| IBIS file 3599z.ibs created by s2ibis2 version 1.1
| North Carolina State University Electronics Research Laboratory  1995
[IBIS ver]   2.1
[File name]   idt70v3599dr.ibs
[File Rev]   2.0
|1.0 : Original Version - Wei-Ling Chang
|2.0 : Replaced I/O and Input models with 70V659 ADC models - S.Kashyap 06/30/04
|3.0:  Modified for DR package - T. Hiatt 4/27/06
[Source]   Integrated Device Technology, Inc.
[Notes]   1.Temperatures: typ=25C, min=100C, max=0C 2.RRmp rates based
   on 50 ohm load. 3. Both inpad and iopad have 2 models each.
   (JTAG pins have one model.)
   iopad: standard 3.3V I/O model
   inpad: standard 3.3V input pad model
   iopad25: For 2.5V I/O supply
   inpad25: For 2.5V I/O supply.
   To use 2.%V models at any port, use iopad25 and inpad25
   as the model definition in pin defie section of the IBIS
   file.  JTAG pins only have models for 3.3V I/O voltage.
[Disclaimer] Integrated Device Technology, Inc. ("IDT") hereby grants the
   user of this IBIS model a non-exclusive, nontransferable
   license to use this IBIS model under the following terms. The
   user is granted this license only to use the IBIS model and is
   not granted rights to sell, copy (except as needed to run the
   IBIS model), rent, lease or sub-license the IBIS model in
   whole or in part, or in modified form to anyone. The User may
   modify the IBIS model to suit its specific applications, but
   rights to derivative works and such modifications shall belong
   to IDT. This IBIS model is provided on an AS IS" basis and IDT
   makes absolutely no warranty with respect to the information
   contained herein. IDT DISCLAIMS AND CUSTOMER WAIVES ALL
   WARRANTIES, EXPRESS AND IMPLIED, INCLUDING WARRANTIES OF
   MERCHANTABILITY AND FITNESS FOR A PARTICULAR PURPOSE. THE
   ENTIRE RISK AS TO QUALITY AND PERFORMANCE IS WITH THE USER
   ACCORDINGLY, IN NO EVENT SHALL IDT BE LIABLE FOR ANY DIRECT OR
   INDIRECT DAMAGES, WHETHER IN CONTRACT OR TORT, INCLUDING ANY
   LOST PROFITS OR OTHER INCIDENTAL, CONSEQUENTIAL, EXEMPLARY, OR
   PUNITIVE DAMAGES ARISING OUT OF THE USE OR APPLICATION OF THE
   IBIS model. Further, IDT reserves the right to make changes
   without notice to any product herein to improve reliability,
   function, or design. IDT does not convey any license under
   patent rights or any other intellectual property rights,
   including those of third parties. IDT is not obligated to
   provide maintenance or support for the licensed IBIS model.
[Copyright]   Copyright 2004, Integrated Device Technology, Inc. all rights
   reserved
|   Component idt70v3599z
[Component]   idt70v3599z
[Manufacturer]   Integrated Device Technology
[Package]
| TQFP (DR208)
| variable   typ   min   max
R_pkg   100.00m   50.00m   0.30
L_pkg   12.00nH   10.00nH   14.00nH
C_pkg   2.80pF   1.50pF   6.00pF
[Pin]  signal_name   model_name   R_pin   L_pin   C_pin
1   io19l   iopad
2   io19r   iopad
3   io20l   iopad
4   io20r   iopad
5   VDDQ   POWER
6   GND   GND
7   io21l   iopad
8   io21r   iopad
9   io22l   iopad
10   io22r   iopad
11   VDDQ   POWER
12   GND   GND
13   io23l   iopad
14   io23r   iopad
15   io24l   iopad
16   io24r   iopad
17   VDDQ   POWER
18   GND   GND
19   io25l   iopad
20   io25r   iopad
21   io26l   iopad
22   io26r   iopad
23   VDDQ   POWER
24   GND   GND
25   VDD   POWER
26   VDD   POWER
27   GND   GND
28   GND   GND
29   VDDQ   POWER
30   GND   GND
31   io27r   iopad
32   io27l   iopad
33   io28r   iopad
34   io28l   iopad
35   VDDQ   POWER
36   GND   GND
37   io29r   iopad
38   io29l   iopad
39   io30r   iopad
40   io30l   iopad
41   VDDQ   POWER
42   GND   GND
43   io31r   iopad
44   io31l   iopad
45   io32r   iopad
46   io32l   iopad
47   VDDQ   POWER
48   GND   GND
49   io33r   iopad
50   io33l   iopad
51   io34r   iopad
52   io34l   iopad
53   GND   GND
54   VDDQ   POWER
55   io35r   iopad
56   io35l   iopad
57   plftr#   inpad
64   a16r   inpad
65   a15r   inpad
66   a14r   inpad
67   a13r   inpad
68   a12r   inpad
69   a11r   inpad
70   a10r   inpad
71   a9r   inpad
72   a8r   inpad
73   a7r   inpad
74   be3r#   inpad
75   be2r#   inpad
76   be1r#   inpad
77   be0r#   inpad
78   ce1r   inpad
79   ce0r   inpad
80   VDD   POWER
81   VDD   POWER
82   GND   GND
83   GND   GND
84   clkr   inpad
85   oe#   inpad
86   rwr#   inpad
87   adsr#   inpad
88   cntenr#   inpad
89   repeatr#   inpad
90   a6r   inpad
91   a5r   inpad
92   a4r   inpad
93   a3r   inpad
94   a2r   inpad
95   a1r   inpad
96   a0r   inpad
97   VDD   POWER
98   GND   GND
99   GND   GND
100   optr   inpad
101   io0l   iopad
102   io0r   iopad
103   VDDQ   POWER
104   GND   GND
105   io1l   iopad
106   io1r   iopad
107   io2l   iopad
108   io2r   iopad
109   VDDQ   POWER
110   GND   GND
111   io3l   iopad
112   io3r   iopad
113   io4l   iopad
114   io4r   iopad
115   VDDQ   POWER
116   GND   GND
117   io5l   iopad
118   io5r   iopad
119   io6l   iopad
120   io6r   iopad
121   VDDQ   POWER
122   GND   GND
123   io7l   iopad
124   io7r   iopad
125   io8l   iopad
126   io8r   iopad
127   VDDQ   POWER
128   GND   GND
129   GND   GND
130   GND   GND
131   VDD   POWER
132   VDD   POWER
133   VDDQ   POWER
134   GND   GND
135   io9r   iopad
136   io9l   iopad
137   io10r   iopad
138   io10l   iopad
139   VDDQ   POWER
140   GND   GND
141   io11r   iopad
142   io11l   iopad
143   io12r   iopad
144   io12l   iopad
145   VDDQ   POWER
146   GND   GND
147   io13r   iopad
148   io13l   iopad
149   io14r   iopad
150   io14l   iopad
151   VDDQ   POWER
152   GND   GND
153   io15r   iopad
154   io15l   iopad
155   io16r   iopad
156   io16l   iopad
157   GND   GND
158   VDDQ   POWER
159   io17r   iopad
160   io17l   iopad
161   optl   inpad
162   GND   GND
163   VDD   POWER
164   VDD   POWER
165   a0l   inpad
166   a1l   inpad
167   a2l   inpad
168   a3l   inpad
169   a4l   inpad
170   a5l   inpad
171   a6l   inpad
172   repeatl#   inpad
173   cntenl#   inpad
174   adsl#   inpad
175   rwl#   inpad
176   oel#   inpad
177   clkl   inpad
178   GND   GND
179   GND   GND
180   VDD   POWER
181   VDD   POWER
182   ce0l#   inpad
183   ce1l   inpad
184   be0l#   inpad
185   be1l#   inpad
186   be2l#   inpad
187   be3l#   inpad
188   a7l   inpad
189   a8l   inpad
190   a9l   inpad
191   a10l   inpad
192   a11l   inpad
193   a12l   inpad
194   a13l   inpad
195   a14l   inpad
196   a15l   inpad
197   a16l   inpad
203   plftl#   inpad
204   test/GND   GND
205   io18l   iopad
206   io18r   iopad
207   VDDQ   POWER
208   GND   GND
| in   in   dummy_model
| oe   oe   dummy_model
[Pin Mapping]  pulldown_ref   pullup_ref   gnd_clamp_ref   power_clamp_ref
1   EXTGND   EXTVDDQ   EXTGND   EXTVDD
2	EXTGND   EXTVDDQ   EXTGND   EXTVDD
3	EXTGND   EXTVDDQ   EXTGND   EXTVDD
4	EXTGND   EXTVDDQ   EXTGND   EXTVDD
5	NC   EXTVDDQ
6	EXTGND   NC
7	EXTGND   EXTVDDQ   EXTGND   EXTVDD
8	EXTGND   EXTVDDQ   EXTGND   EXTVDD
9	EXTGND   EXTVDDQ   EXTGND   EXTVDD
10	EXTGND   EXTVDDQ   EXTGND   EXTVDD
11	NC   EXTVDDQ
12	EXTGND   NC
13	EXTGND   EXTVDDQ   EXTGND   EXTVDD
14	EXTGND   EXTVDDQ   EXTGND   EXTVDD
15	EXTGND   EXTVDDQ   EXTGND   EXTVDD
16	EXTGND   EXTVDDQ   EXTGND   EXTVDD
17	NC   EXTVDDQ
18	EXTGND   NC
19	EXTGND   EXTVDDQ   EXTGND   EXTVDD
20	EXTGND   EXTVDDQ   EXTGND   EXTVDD
21	EXTGND   EXTVDDQ   EXTGND   EXTVDD
22	EXTGND   EXTVDDQ   EXTGND   EXTVDD
23	NC   EXTVDDQ
24	EXTGND   NC
25	NC   EXTVDD
26	NC   EXTVDD
27	EXTGND   NC
28	EXTGND   NC
29	NC   EXTVDDQ
30	EXTGND   NC
31	EXTGND   EXTVDDQ   EXTGND   EXTVDD
32	EXTGND   EXTVDDQ   EXTGND   EXTVDD
33	EXTGND   EXTVDDQ   EXTGND   EXTVDD
34	EXTGND   EXTVDDQ   EXTGND   EXTVDD
35	NC   EXTVDDQ
36	EXTGND   NC
37	EXTGND   EXTVDDQ   EXTGND   EXTVDD
38	EXTGND   EXTVDDQ   EXTGND   EXTVDD
39	EXTGND   EXTVDDQ   EXTGND   EXTVDD
40	EXTGND   EXTVDDQ   EXTGND   EXTVDD
41	NC   EXTVDDQ
42	EXTGND   NC
43	EXTGND   EXTVDDQ   EXTGND   EXTVDD
44	EXTGND   EXTVDDQ   EXTGND   EXTVDD
45	EXTGND   EXTVDDQ   EXTGND   EXTVDD
46	EXTGND   EXTVDDQ   EXTGND   EXTVDD
47	NC   EXTVDDQ
48	EXTGND   NC
49	EXTGND   EXTVDDQ   EXTGND   EXTVDD
50	EXTGND   EXTVDDQ   EXTGND   EXTVDD
51	EXTGND   EXTVDDQ   EXTGND   EXTVDD
52	EXTGND   EXTVDDQ   EXTGND   EXTVDD
53	EXTGND   NC
54	NC   EXTVDDQ
55	EXTGND   EXTVDDQ   EXTGND   EXTVDD
56	EXTGND   EXTVDDQ   EXTGND   EXTVDD
57	EXTGND   EXTVDDQ   EXTGND   EXTVDD
64	EXTGND   EXTVDDQ   EXTGND   EXTVDD
65	EXTGND   EXTVDDQ   EXTGND   EXTVDD
66	EXTGND   EXTVDDQ   EXTGND   EXTVDD
67	EXTGND   EXTVDDQ   EXTGND   EXTVDD
68	EXTGND   EXTVDDQ   EXTGND   EXTVDD
69	EXTGND   EXTVDDQ   EXTGND   EXTVDD
70	EXTGND   EXTVDDQ   EXTGND   EXTVDD
71	EXTGND   EXTVDDQ   EXTGND   EXTVDD
72	EXTGND   EXTVDDQ   EXTGND   EXTVDD
73	EXTGND   EXTVDDQ   EXTGND   EXTVDD
74	EXTGND   EXTVDDQ   EXTGND   EXTVDD
75	EXTGND   EXTVDDQ   EXTGND   EXTVDD
76	EXTGND   EXTVDDQ   EXTGND   EXTVDD
77	EXTGND   EXTVDDQ   EXTGND   EXTVDD
78	EXTGND   EXTVDDQ   EXTGND   EXTVDD
79	EXTGND   EXTVDDQ   EXTGND   EXTVDD
80	NC   EXTVDD
81	NC   EXTVDD
82	EXTGND   NC
83	EXTGND   NC
84	EXTGND   EXTVDDQ   EXTGND   EXTVDD
85	EXTGND   EXTVDDQ   EXTGND   EXTVDD
86	EXTGND   EXTVDDQ   EXTGND   EXTVDD
87	EXTGND   EXTVDDQ   EXTGND   EXTVDD
88	EXTGND   EXTVDDQ   EXTGND   EXTVDD
89	EXTGND   EXTVDDQ   EXTGND   EXTVDD
90	EXTGND   EXTVDDQ   EXTGND   EXTVDD
91	EXTGND   EXTVDDQ   EXTGND   EXTVDD
92	EXTGND   EXTVDDQ   EXTGND   EXTVDD
93	EXTGND   EXTVDDQ   EXTGND   EXTVDD
94	EXTGND   EXTVDDQ   EXTGND   EXTVDD
95	EXTGND   EXTVDDQ   EXTGND   EXTVDD
96	EXTGND   EXTVDDQ   EXTGND   EXTVDD
97	NC   EXTVDD
98	EXTGND   NC
99	EXTGND   NC
100	EXTGND   EXTVDDQ   EXTGND   EXTVDD
101	EXTGND   EXTVDDQ   EXTGND   EXTVDD
102	EXTGND   EXTVDDQ   EXTGND   EXTVDD
103	NC   EXTVDDQ
104	EXTGND   NC
105	EXTGND   EXTVDDQ   EXTGND   EXTVDD
106	EXTGND   EXTVDDQ   EXTGND   EXTVDD
107	EXTGND   EXTVDDQ   EXTGND   EXTVDD
108	EXTGND   EXTVDDQ   EXTGND   EXTVDD
109	NC   EXTVDDQ
110	EXTGND   NC
111	EXTGND   EXTVDDQ   EXTGND   EXTVDD
112	EXTGND   EXTVDDQ   EXTGND   EXTVDD
113	EXTGND   EXTVDDQ   EXTGND   EXTVDD
114	EXTGND   EXTVDDQ   EXTGND   EXTVDD
115	NC   EXTVDDQ
116	EXTGND   NC
117	EXTGND   EXTVDDQ   EXTGND   EXTVDD
118	EXTGND   EXTVDDQ   EXTGND   EXTVDD
119	EXTGND   EXTVDDQ   EXTGND   EXTVDD
120	EXTGND   EXTVDDQ   EXTGND   EXTVDD
121	NC   EXTVDDQ
122	EXTGND   NC
123	EXTGND   EXTVDDQ   EXTGND   EXTVDD
124	EXTGND   EXTVDDQ   EXTGND   EXTVDD
125	EXTGND   EXTVDDQ   EXTGND   EXTVDD
126	EXTGND   EXTVDDQ   EXTGND   EXTVDD
127	NC   EXTVDDQ
128	EXTGND   NC
129	EXTGND   NC
130	EXTGND   NC
131	NC   EXTVDD
132	NC   EXTVDD
133	NC   EXTVDDQ
134	EXTGND   NC
135	EXTGND   EXTVDDQ   EXTGND   EXTVDD
136	EXTGND   EXTVDDQ   EXTGND   EXTVDD
137	EXTGND   EXTVDDQ   EXTGND   EXTVDD
138	EXTGND   EXTVDDQ   EXTGND   EXTVDD
139	NC   EXTVDDQ
140	EXTGND   NC
141	EXTGND   EXTVDDQ   EXTGND   EXTVDD
142	EXTGND   EXTVDDQ   EXTGND   EXTVDD
143	EXTGND   EXTVDDQ   EXTGND   EXTVDD
144	EXTGND   EXTVDDQ   EXTGND   EXTVDD
145	NC   EXTVDDQ
146	EXTGND   NC
147	EXTGND   EXTVDDQ   EXTGND   EXTVDD
148	EXTGND   EXTVDDQ   EXTGND   EXTVDD
149	EXTGND   EXTVDDQ   EXTGND   EXTVDD
150	EXTGND   EXTVDDQ   EXTGND   EXTVDD
151	NC   EXTVDDQ
152	EXTGND   NC
153	EXTGND   EXTVDDQ   EXTGND   EXTVDD
154	EXTGND   EXTVDDQ   EXTGND   EXTVDD
155	EXTGND   EXTVDDQ   EXTGND   EXTVDD
156	EXTGND   EXTVDDQ   EXTGND   EXTVDD
157	EXTGND   NC
158	NC   EXTVDDQ
159	EXTGND   EXTVDDQ   EXTGND   EXTVDD
160	EXTGND   EXTVDDQ   EXTGND   EXTVDD
161	EXTGND   EXTVDDQ   EXTGND   EXTVDD
162	EXTGND   NC
163	NC   EXTVDD
164	NC   EXTVDD
165	EXTGND   EXTVDDQ   EXTGND   EXTVDD
166	EXTGND   EXTVDDQ   EXTGND   EXTVDD
167	EXTGND   EXTVDDQ   EXTGND   EXTVDD
168	EXTGND   EXTVDDQ   EXTGND   EXTVDD
169	EXTGND   EXTVDDQ   EXTGND   EXTVDD
170	EXTGND   EXTVDDQ   EXTGND   EXTVDD
171	EXTGND   EXTVDDQ   EXTGND   EXTVDD
172	EXTGND   EXTVDDQ   EXTGND   EXTVDD
173	EXTGND   EXTVDDQ   EXTGND   EXTVDD
174	EXTGND   EXTVDDQ   EXTGND   EXTVDD
175	EXTGND   EXTVDDQ   EXTGND   EXTVDD
176	EXTGND   EXTVDDQ   EXTGND   EXTVDD
177	EXTGND   EXTVDDQ   EXTGND   EXTVDD
178	EXTGND   NC
179	EXTGND   NC
180	NC   EXTVDD
181	NC   EXTVDD
182	EXTGND   EXTVDDQ   EXTGND   EXTVDD
183	EXTGND   EXTVDDQ   EXTGND   EXTVDD
184	EXTGND   EXTVDDQ   EXTGND   EXTVDD
185	EXTGND   EXTVDDQ   EXTGND   EXTVDD
186	EXTGND   EXTVDDQ   EXTGND   EXTVDD
187	EXTGND   EXTVDDQ   EXTGND   EXTVDD
188	EXTGND   EXTVDDQ   EXTGND   EXTVDD
189	EXTGND   EXTVDDQ   EXTGND   EXTVDD
190	EXTGND   EXTVDDQ   EXTGND   EXTVDD
191	EXTGND   EXTVDDQ   EXTGND   EXTVDD
192	EXTGND   EXTVDDQ   EXTGND   EXTVDD
193	EXTGND   EXTVDDQ   EXTGND   EXTVDD
194	EXTGND   EXTVDDQ   EXTGND   EXTVDD
195	EXTGND   EXTVDDQ   EXTGND   EXTVDD
196	EXTGND   EXTVDDQ   EXTGND   EXTVDD
197	EXTGND   EXTVDDQ   EXTGND   EXTVDD
203	EXTGND   EXTVDDQ   EXTGND   EXTVDD
204	EXTGND   NC
205	EXTGND   EXTVDDQ   EXTGND   EXTVDD
206	EXTGND   EXTVDDQ   EXTGND   EXTVDD
207	NC   EXTVDDQ
208	EXTGND   NC
| Models and submodels in the file (5): iopad (I/O), inpad (Input), inpadbs (Input), iopad25 (I/O), inpad25 (Input)
